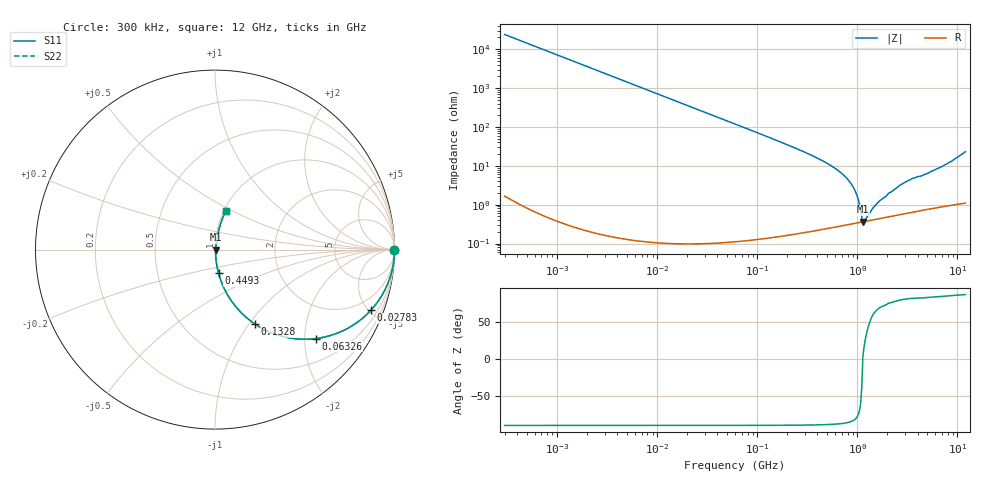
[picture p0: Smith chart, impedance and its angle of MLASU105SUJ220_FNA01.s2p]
! MLASU105SUJ220_FNA01  S-PARAMETER MODEL  ( General Type )
! Model Generated by TAIYO YUDEN Corporation (http://www.ty-top.com)
! Version 3.0
! TAIYO YUDEN Control No. 120810
! Copyright(c) 2003 TAIYO YUDEN CO.,LTD. All Rights Reserved.
! Product Description (link to TY-COMPAS)
! https://ds.yuden.co.jp/TYCOMPAS/or/detail?pn=MLASU105SUJ220JFNA01&u=M
! Products Name : Multilayer Ceramic Capacitors
! Characteristics :
!  Capacitance : 22 pF , Rated Voltage : 50V , TCC : UJ / U2J
!  Case Size : 1.0 x 0.5 / 0.039 x 0.02 [mm/inch] , Thickness : 0.5 / 0.02 [mm/inch]
!  (Conditions: Temperature = 25 degC , DC Bias Current/Voltage = 0A / 0V)
! External Node Assignments :
!  1  o---| |---o  2
! GND o---------o GND
! Frequency Range : 0.3MHz  -  12000MHz  [ 401 STEP ]
# MHz S RI R 50
! Freq[MHz].  S11 Real  S11 Imag  S21 Real  S21 Imag  S12 Real  S12 Imag  S22 Real  S22 Imag
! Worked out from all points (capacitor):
!   401 points, 300 kHz to 12 GHz, reference 50 ohm
!   read as one part in series: C = 22.2 pF near 316.3 kHz
!   lowest |Z| = 363 mohm at 1.136 GHz (marker M1)
!   series resonance near 1.134 GHz, so ESL is about 890 pH
!   S11 on the Smith chart (normalised r, x): 300 kHz: open; 27.83 MHz: 1.00, -5.15; 63.26 MHz: 1.00, -2.26; 132.8 MHz: 1.00, -1.07; 449.3 MHz: 1.00, -0.27; 12 GHz: 1.02, +0.46
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0.3  1 -0.00418  1.78e-05 0.00418  1.78e-05 0.00418  1 -0.00418
1.769972  0.9994 -0.0247  0.00061 0.0247  0.00061 0.0247  0.9994 -0.0247
10.44266  0.9792 -0.1426  0.0208 0.1426  0.0208 0.1426  0.9792 -0.1426
27.82928  0.8689 -0.3373  0.1311 0.3373  0.1311 0.3373  0.8689 -0.3373
60  0.5869 -0.4919  0.4131 0.4919  0.4131 0.4919  0.5869 -0.4919
63.26471  0.5609 -0.4958  0.4391 0.4958  0.4391 0.4958  0.5609 -0.4958
89.27472  0.3895 -0.4869  0.6105 0.4869  0.6105 0.4869  0.3895 -0.4869
132.8329  0.2216 -0.414  0.7784 0.414  0.7784 0.414  0.2216 -0.414
208.3979  0.1008 -0.2986  0.8992 0.2986  0.8992 0.2986  0.1008 -0.2986
353.9943  0.0342 -0.1762  0.9658 0.1762  0.9658 0.1762  0.0342 -0.1762
449.3064  0.02 -0.1315  0.98 0.1315  0.98 0.1315  0.02 -0.1315
651.0506  0.00811 -0.073  0.9919 0.073  0.9919 0.073  0.00811 -0.073
848.5281  0.00449 -0.0368  0.9955 0.0368  0.9955 0.0368  0.00449 -0.0368
968.706  0.00373 -0.0198  0.9963 0.0198  0.9963 0.0198  0.00373 -0.0198
1021.415  0.0036 -0.013  0.9964 0.013  0.9964 0.013  0.0036 -0.013
1135.593  0.00361 0.000188  0.9964 -0.000188  0.9964 -0.000188  0.00361 0.000188
1197.383  0.00371 0.00179  0.9963 -0.00179  0.9963 -0.00179  0.00371 0.00179
1519.776  0.00426 0.00871  0.9957 -0.00871  0.9957 -0.00871  0.00426 0.00871
2088.533  0.00529 0.0194  0.9947 -0.0194  0.9947 -0.0194  0.00529 0.0194
3026.31  0.0073 0.0373  0.9927 -0.0373  0.9927 -0.0373  0.0073 0.0373
6699.894  0.0164 0.0881  0.9836 -0.0881  0.9836 -0.0881  0.0164 0.0881
12000  0.0594 0.2137  0.9406 -0.2137  0.9406 -0.2137  0.0594 0.2137
